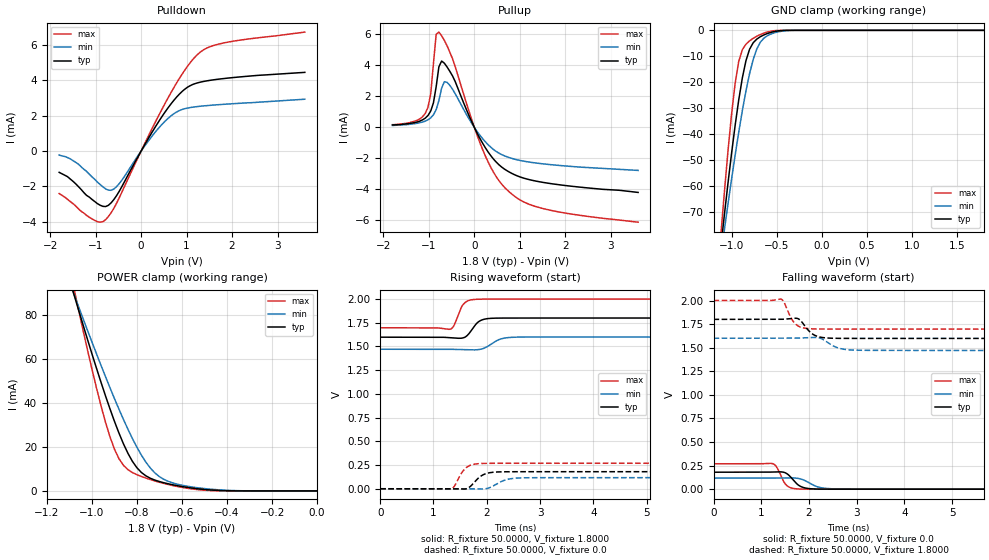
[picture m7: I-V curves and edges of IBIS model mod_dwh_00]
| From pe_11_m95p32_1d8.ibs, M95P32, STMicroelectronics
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|   Model mod_dwh_00
[Model]   mod_dwh_00
Model_type I/O
Polarity   Non-Inverting
Enable   Active-High
Vinl   =   0.540V
Vinh   =   1.260V
Vmeas  =   0.900V
Cref   =   30.0pF
C_comp   1.630pF   1.607pF   1.683pF
[Model Spec]
Vinl   0.540V  0.480V  0.600V  | <- for Vcc = 1.8V, 1.6V, 2.0V
Vinh   1.260V  1.120V  1.400V  | <- for Vcc = 1.8V, 1.6V, 2.0V
Vmeas  0.900V  0.800V  1.000V  | <- for Vcc = 1.8V, 1.6V, 2.0V
[Temperature Range]  25.0000   0.1050k   -40.0000
[Voltage Range]   1.8000V   1.6000V   2.0000V
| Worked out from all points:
|   slope of the pulldown table from 0 to 0.27 V, typ, clamps not added: 227 ohm
|   slope of the pullup table from 0 to 0.27 V, typ, clamps not added: 188 ohm
|   GND clamp passes 1 mA (typ) near -0.58 V on its own axis
|   POWER clamp passes 1 mA (typ) near -0.53 V on its own axis
|   rising waveform, R_fixture 50.0000, V_fixture 1.8000: 20-80 % time 173ps typ, 233ps min, 138ps max; typ from 1.6 V to 1.8 V
|   rising waveform, R_fixture 50.0000, V_fixture 0.0: 20-80 % time 207ps typ, 255ps min, 179ps max; typ from 0 V to 0.18 V
|   falling waveform, R_fixture 50.0000, V_fixture 0.0: 20-80 % time 213ps typ, 282ps min, 161ps max; typ from 0.18 V to 0 V
|   falling waveform, R_fixture 50.0000, V_fixture 1.8000: 20-80 % time 224ps typ, 277ps min, 188ps max; typ from 1.8 V to 1.6 V
[Pulldown]
|Voltage   I(typ)   I(min)   I(max)
-1.8V     -1.2mA     -220uA     -2.4mA
-1.38V    -2mA       -730uA     -3.26mA
-1.02V    -2.85mA    -1.59mA    -3.92mA
-840mV    -3.125mA   -2.02mA    -3.993mA
-660mV    -2.931mA   -2.218mA   -3.494mA
-540mV    -2.525mA   -2.014mA   -2.958mA
240mV     1.064mA    846.5uA    1.267mA
660mV     2.681mA    2.001mA    3.324mA
960mV     3.505mA    2.404mA    4.584mA
1.26V     3.879mA    2.53mA     5.517mA
1.86V     4.122mA    2.659mA    6.148mA
3.6V      4.46mA     2.94mA     6.74mA
[Pullup]
|Voltage   I(typ)   I(min)   I(max)
-1.8V     160uA      130uA      180uA
-1.08V    602uA      410uA      907uA
-960mV    1.058mA    620uA      2.158mA
-900mV    1.592mA    816uA      4.119mA
-840mV    2.634mA    1.149mA    6.013mA
-780mV    3.914mA    1.734mA    6.153mA
-660mV    4.145mA    2.953mA    5.618mA
-600mV    3.902mA    2.912mA    5.267mA
180mV     -1.012mA   -717.7uA   -1.417mA
720mV     -2.795mA   -1.896mA   -4.031mA
1.5V      -3.538mA   -2.344mA   -5.223mA
3.6V      -4.19mA    -2.77mA    -6.11mA
[GND_clamp]
|Voltage   I(typ)   I(min)   I(max)
-1.8V     -319.7mA   -274.4mA   -407.3mA
-1.12V    -83.64mA   -87.01mA   -79.32mA
-1.08V    -71.08mA   -76.85mA   -62.45mA
-1V       -47.38mA   -57.28mA   -32.33mA
-960mV    -36.55mA   -47.99mA   -20.38mA
-920mV    -26.73mA   -39.15mA   -11.92mA
-840mV    -11.67mA   -23.32mA   -5.34mA
-760mV    -4.801mA   -11.23mA   -3.081mA
-720mV    -3.384mA   -7.183mA   -2.279mA
-640mV    -1.748mA   -2.99mA    -1.048mA
-440mV    -85.93uA   -314uA     -8.035uA
1.8V      367pA      1.678uA    95.55pA
[POWER_clamp]
|Voltage   I(typ)   I(min)   I(max)
-1.8V     354.3mA    299.2mA    462.7mA
-1.08V    89.41mA    89.52mA    92.12mA
-1.06V    82.53mA    84.01mA    82.65mA
-980mV    55.86mA    62.44mA    46.9mA
-920mV    37.35mA    46.96mA    24.63mA
-880mV    26.31mA    37.17mA    14.66mA
-840mV    17.07mA    28.03mA    9.669mA
-800mV    10.51mA    19.82mA    7.37mA
-740mV    5.731mA    10.32mA    5.151mA
-640mV    2.77mA     3.598mA    2.408mA
-420mV    154.7uA    391.9uA    29.01uA
0V        367pA      19.37nA    169pA
[Ramp]
| variable   typ   min   max
dV/dt_r  0.1078/0.2627n   70.1335m/0.3855n   0.1613/0.2256n
dV/dt_f  0.1212/0.3422n   77.4600m/0.5045n   0.1817/0.2879n
R_load = 50.0000
[Rising Waveform]
R_fixture= 50.0000
V_fixture= 1.8000
V_fixture_min= 1.6000
V_fixture_max= 2.0000
|time   V(typ)   V(min)   V(max)
0s        1.598V     1.471V     1.697V
1.312ns   1.593V     1.471V     1.682V
1.392ns   1.589V     1.469V     1.73V
1.504ns   1.587V     1.467V     1.89V
1.568ns   1.593V     1.466V     1.95V
1.792ns   1.732V     1.464V     1.997V
1.984ns   1.791V     1.491V     2V
2.24ns    1.799V     1.575V     2V
2.512ns   1.8V       1.598V     2V
8ns       1.8V       1.6V       2V
[Rising Waveform]
R_fixture= 50.0000
V_fixture= 0.0
V_fixture_min= 0.0
V_fixture_max= 0.0
|time   V(typ)   V(min)   V(max)
0s        6.626nV    816.4nV    1.089nV
1.336ns   88.47uV    172.2uV    -1.733mV
1.384ns   -220.2uV   182.8uV    20.7mV
1.528ns   -3.099mV   122.3uV    167.1mV
1.608ns   -1.582mV   -63.13uV   219.5mV
1.864ns   122.9mV    -2.68mV    265.2mV
2.088ns   172mV      19.92mV    268.4mV
2.344ns   179mV      91.64mV    268.8mV
2.632ns   179.7mV    114.2mV    268.8mV
8ns       179.7mV    116.9mV    268.8mV
[Falling Waveform]
R_fixture= 50.0000
V_fixture= 0.0
V_fixture_min= 0.0
V_fixture_max= 0.0
|time   V(typ)   V(min)   V(max)
0s        179.7mV    116.9mV    268.8mV
1.232ns   181.7mV    116.9mV    271.5mV
1.328ns   183.5mV    117.7mV    230.5mV
1.456ns   180.9mV    118.8mV    93.8mV
1.52ns    169.7mV    119.4mV    46.24mV
1.76ns    50.46mV    115.5mV    2.665mV
1.92ns    12.7mV     90.01mV    397.6uV
2.192ns   901uV      22.64mV    19.42uV
2.544ns   32.53uV    2.455mV    1.419uV
8ns       241.8nV    983nV      336.1nV
[Falling Waveform]
R_fixture= 50.0000
V_fixture= 1.8000
V_fixture_min= 1.6000
V_fixture_max= 2.0000
|time   V(typ)   V(min)   V(max)
0s        1.8V       1.6V       2V
1.424ns   1.8V       1.6V       2.013V
1.472ns   1.802V     1.6V       1.987V
1.696ns   1.812V     1.6V       1.762V
1.808ns   1.795V     1.602V     1.721V
2ns       1.677V     1.606V     1.701V
2.272ns   1.608V     1.593V     1.698V
2.592ns   1.599V     1.5V       1.697V
2.928ns   1.598V     1.474V     1.697V
8ns       1.598V     1.471V     1.697V
